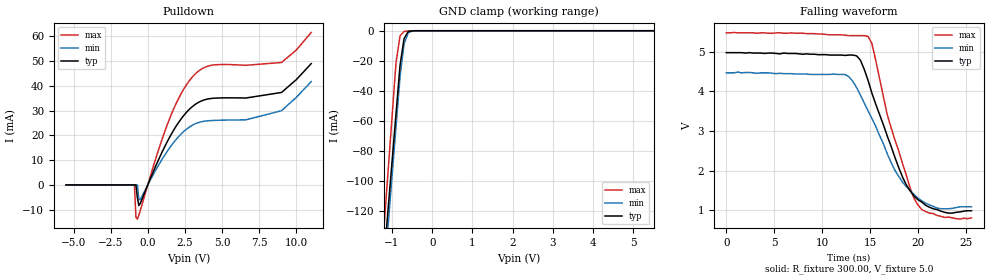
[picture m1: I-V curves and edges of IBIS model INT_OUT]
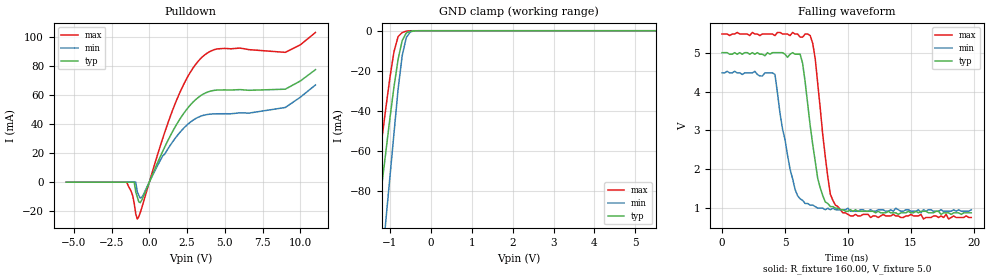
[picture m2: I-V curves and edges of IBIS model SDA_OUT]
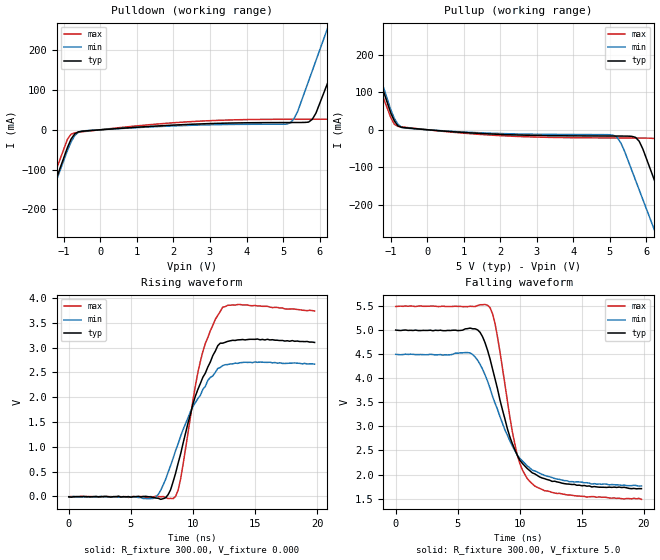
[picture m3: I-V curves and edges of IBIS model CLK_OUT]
| IBIS file 8564nb5v.ibs
[IBIS ver]   3.2
[File name]   8564nb5v.ibs
[File Rev]   1.0
[Date]   Jan 22, 2008
[Source]   This file orginated at EPSON TOYOCOM Corp.
[Copyright]   Copyright EPSON TOYOCOM Corp. 2008
|   Component 8564nb5v
[Component]   8564nb5v
[Manufacturer]   EPSON TOYOCOM
[Package]
| variable   typ   min   max
R_pkg   87m   NA   NA
L_pkg   10nH   NA   NA
C_pkg   206fF   NA   NA
[Pin]  signal_name   model_name   R_pin   L_pin   C_pin
1   /INT   INT_OUT
2   GND   GND
|3   GND
|4   NC
5   SDA   SDA_OUT
6   SCL   SCL_IN
7   CLKOUT   CLK_OUT
8   VDD   POWER
9   CLKOE   OE_IN
|10   NC
|11   NC
|12   NC
|13   NC
|14   NC
|15   NC
|16   NC
|17   NC
|18   NC
|19   NC
|20   NC
|21   NC
|22   NC
5T   SDA   SDA_IN
| Models and submodels in the file (6): INT_OUT (Open_drain), SDA_OUT (Open_drain), CLK_OUT (Output), SCL_IN (Input), OE_IN (Input), SDA_IN (Input)
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|   Model OUTPUT
[Model]   INT_OUT
Model_type   Open_drain
Polarity   Non-Inverting
C_comp   5pF   5pF   5pF
[Temperature Range]   25.00   85.00   -40.000
[Voltage Range]   5.0V   4.5V   5.5V
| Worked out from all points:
|   slope of the pulldown table from 0 to 0.75 V, typ, clamps not added: 71.5 ohm
|   GND clamp passes 1 mA (typ) near -0.61 V on its own axis
|   falling waveform, R_fixture 300.00, V_fixture 5.0: 20-80 % time 3.58ns typ, 4.02ns min, 3.16ns max; typ from 4.98 V to 0.99 V
[Pulldown]
| voltage   I(typ)   I(min)   I(max)
-5.5V     0A         0A         0A
-900mV    0A         0A         0A
-800mV    0A         0A         -13.02mA
-700mV    -5.27mA    0A         -13.77mA
-600mV    -8.31mA    -5.95mA    -12.17mA
-500mV    -7.37mA    -5.89mA    -10.2mA
1.5V      19.59mA    15.21mA    27.22mA
2.3V      27.1mA     20.9mA     37.45mA
3.1V      32.08mA    24.41mA    44.2mA
4.4V      34.97mA    26.01mA    48.4mA
9V        37.31mA    29.95mA    49.41mA
11V       48.95mA    41.69mA    61.52mA
[GND_clamp]
| voltage   I(typ)   I(min)   I(max)
-5.5V     -1.538A    -1.601A    -1.706A
-1.2V     -151.9mA   -164mA     -131.1mA
-1.1V     -119.6mA   -130.6mA   -94.45mA
-1V       -87.39mA   -97.2mA    -57.83mA
-900mV    -55.16mA   -63.79mA   -21.21mA
-800mV    -22.93mA   -30.38mA   -3.34mA
-700mV    -5.21mA    -8.93mA    -540uA
-600mV    -650uA     -1.42mA    -90uA
-500mV    -70uA      -140uA     -10uA
5.5V      0A         0A         0A
[Ramp]
| variable   typ   min   max
dV/dt_r 2.59/8.4n   2.23/8.0n   2.99/8.4n
dV/dt_f 2.43/4.0n   2.07/4.4n   2.82/3.6n
R_load = 300.00
[Falling Waveform]
R_fixture = 300.00
V_fixture = 5.0
V_fixture_min = 4.5
V_fixture_max = 5.5
| time   V(typ)   V(min)   V(max)
0s        4.98V      4.47V      5.48V
12.4ns    4.91V      4.43V      5.42V
13.6ns    4.9V       4.1V       5.41V
14.8ns    4.28V      3.51V      5.39V
15.2ns    3.96V      3.32V      5.21V
16.8ns    2.88V      2.43V      3.42V
17.6ns    2.34V      2.01V      2.78V
19.6ns    1.36V      1.4V       1.3V
21.2ns    1.08V      1.14V      930mV
25.6ns    990mV      1.09V      810mV
[Model]   SDA_OUT
Model_type   Open_drain
Polarity   Non-Inverting
C_comp   5pF   5pF   5pF
[Temperature Range]   25.00   85.00   -40.000
[Voltage Range]   5.0V   4.5V   5.5V
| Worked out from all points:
|   slope of the pulldown table from 0 to 0.75 V, typ, clamps not added: 41.3 ohm
|   GND clamp passes 1 mA (typ) near -0.59 V on its own axis
|   falling waveform, R_fixture 160.00, V_fixture 5.0: 20-80 % time 1.02ns typ, 1.2ns min, 949ps max; typ from 5 V to 0.88 V
[Pulldown]
| voltage   I(typ)   I(min)   I(max)
-5.5V     0A         0A         0A
-1.5V     0A         0A         0A
-1V       0A         0A         -14.64mA
-900mV    -6.78mA    0A         -21.87mA
-800mV    -10.08mA   -6.54mA    -25.43mA
-500mV    -12.28mA   -10.58mA   -17.67mA
1.7V      37.93mA    30.09mA    53.88mA
2.6V      51.83mA    40.42mA    73.8mA
3.4V      59.65mA    45.49mA    85.31mA
4.5V      63.53mA    47.17mA    91.92mA
9V        64.12mA    51.5mA     89.52mA
11V       77.6mA     67.04mA    103.2mA
[GND_clamp]
| voltage   I(typ)   I(min)   I(max)
-5.5V     -803.8mA   -1.06A     -733.3mA
-1.5V     -128.2mA   -182.8mA   -102.1mA
-1.4V     -111.3mA   -160.9mA   -86.31mA
-1.3V     -94.44mA   -138.9mA   -70.53mA
-1.1V     -60.66mA   -95.05mA   -38.68mA
-900mV    -27.98mA   -51.17mA   -10.4mA
-800mV    -14.32mA   -29.23mA   -2.93mA
-700mV    -4.92mA    -12.49mA   -900uA
-600mV    -1.08mA    -3.42mA    -200uA
-500mV    -290uA     -530uA     -10uA
-400mV    -60uA      -50uA      0A
5.5V      0A         0A         0A
[Ramp]
| variable   typ   min   max
dV/dt_r 2.47/1.8n   2.21/1.8n   2.69/1.6n
dV/dt_f 2.50/1.0n   2.18/1.0n   2.88/1.0n
R_load = 160.00
[Falling Waveform]
R_fixture = 160.00
V_fixture = 5.0
V_fixture_min = 4.5
V_fixture_max = 5.5
| time   V(typ)   V(min)   V(max)
0s        5V         4.48V      5.48V
4.2ns     5V         4.44V      5.44V
5.4ns     4.96V      2V         5.44V
6.2ns     4.96V      1.24V      5.4V
7ns       3.12V      1.08V      5.44V
7.4ns     2.2V       1.04V      4.84V
7.6ns     1.76V      1V         4.2V
8.6ns     1.04V      960mV      1.36V
9.6ns     960mV      960mV      880mV
19.8ns    880mV      960mV      760mV
[Model]   CLK_OUT
Model_type   Output
Polarity   Non-Inverting
Enable   Active-High
Vmeas =   1.50V
C_comp   1.69pF   1.32pF   1.96pF
[Temperature Range]   25.00   85.00   -40.000
[Voltage Range]   5.0V   4.5V   5.5V
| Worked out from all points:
|   slope of the pulldown table from 0 to 0.75 V, typ, clamps not added: 153 ohm
|   slope of the pullup table from 0 to 0.75 V, typ, clamps not added: 133 ohm
|   rising waveform, R_fixture 300.00, V_fixture 0.000: 20-80 % time 2.24ns typ, 2.7ns min, 1.62ns max; typ from -0.008 V to 3.1 V
|   falling waveform, R_fixture 300.00, V_fixture 5.0: 20-80 % time 2.21ns typ, 2.72ns min, 1.62ns max; typ from 4.99 V to 1.71 V
[Pulldown]
| voltage   I(typ)   I(min)   I(max)
-5.5V     -1.228A    -1.193A    -1.168A
-1.8V     -275.9mA   -275.2mA   -247.5mA
-900mV    -44.38mA   -52.02mA   -23.54mA
-600mV    -5.34mA    -6.13mA    -6.34mA
5.2V      18.13mA    17.33mA    26.3mA
5.8V      26.11mA    148.1mA    26.37mA
6.3V      136.2mA    276mA      26.71mA
6.5V      183.5mA    327.2mA    50.71mA
6.8V      254.5mA    403.9mA    129.6mA
7V        301.8mA    455.1mA    182.3mA
9V        775mA      966.7mA    708.5mA
11V       1.248A     1.478A     1.235A
[Pullup]
| voltage   I(typ)   I(min)   I(max)
-5.5V     1.346A     1.403A     1.205A
-2V       334.2mA    353.6mA    293.3mA
-1.8V     276.3mA    293.6mA    241.2mA
-1V       44.97mA    53.88mA    32.75mA
-700mV    6.35mA     6.24mA     7.64mA
5.1V      -16.83mA   -14.78mA   -21.92mA
5.8V      -30.5mA    -159.9mA   -22.19mA
6.3V      -156.2mA   -288.4mA   -26.34mA
6.7V      -261.6mA   -391.2mA   -117.2mA
7V        -340.6mA   -468.4mA   -194.2mA
9V        -867.4mA   -982.6mA   -707.8mA
11V       -1.394A    -1.497A    -1.221A
[Ramp]
| variable   typ   min   max
dV/dt_r 1.76/2.2n   1.48/2.4n   2.17/1.6n
dV/dt_f 1.99/2.6n   1.66/2.6n   2.42/1.8n
R_load = 300.00
[Rising Waveform]
R_fixture = 300.00
V_fixture = 0.000
| time   V(typ)   V(min)   V(max)
0s        -7.5mV     -12.97mV   -7.97mV
6.8ns     -21.88mV   -42.5mV    -12.97mV
7.8ns     -28.44mV   343mV      -19.84mV
8.4ns     293.8mV    767mV      -45.63mV
9ns       847.8mV    1.209V     341.1mV
10.2ns    2.025V     1.894V     2.233V
10.8ns    2.403V     2.16V      2.923V
12ns      3.04V      2.58V      3.65V
12.4ns    3.09V      2.638V     3.818V
19.8ns    3.105V     2.667V     3.738V
[Falling Waveform]
R_fixture = 300.00
V_fixture = 5.0
V_fixture_min = 4.5
V_fixture_max = 5.5
| time   V(typ)   V(min)   V(max)
0s        4.993V     4.491V     5.482V
6ns       5.034V     4.518V     5.486V
6.8ns     4.945V     4.283V     5.518V
7.4ns     4.575V     3.935V     5.509V
8ns       3.986V     3.483V     5.135V
9.2ns     2.78V      2.698V     3.191V
9.8ns     2.399V     2.404V     2.399V
10.6ns    2.126V     2.18V      1.917V
13ns      1.849V     1.907V     1.609V
19.8ns    1.709V     1.765V     1.488V
